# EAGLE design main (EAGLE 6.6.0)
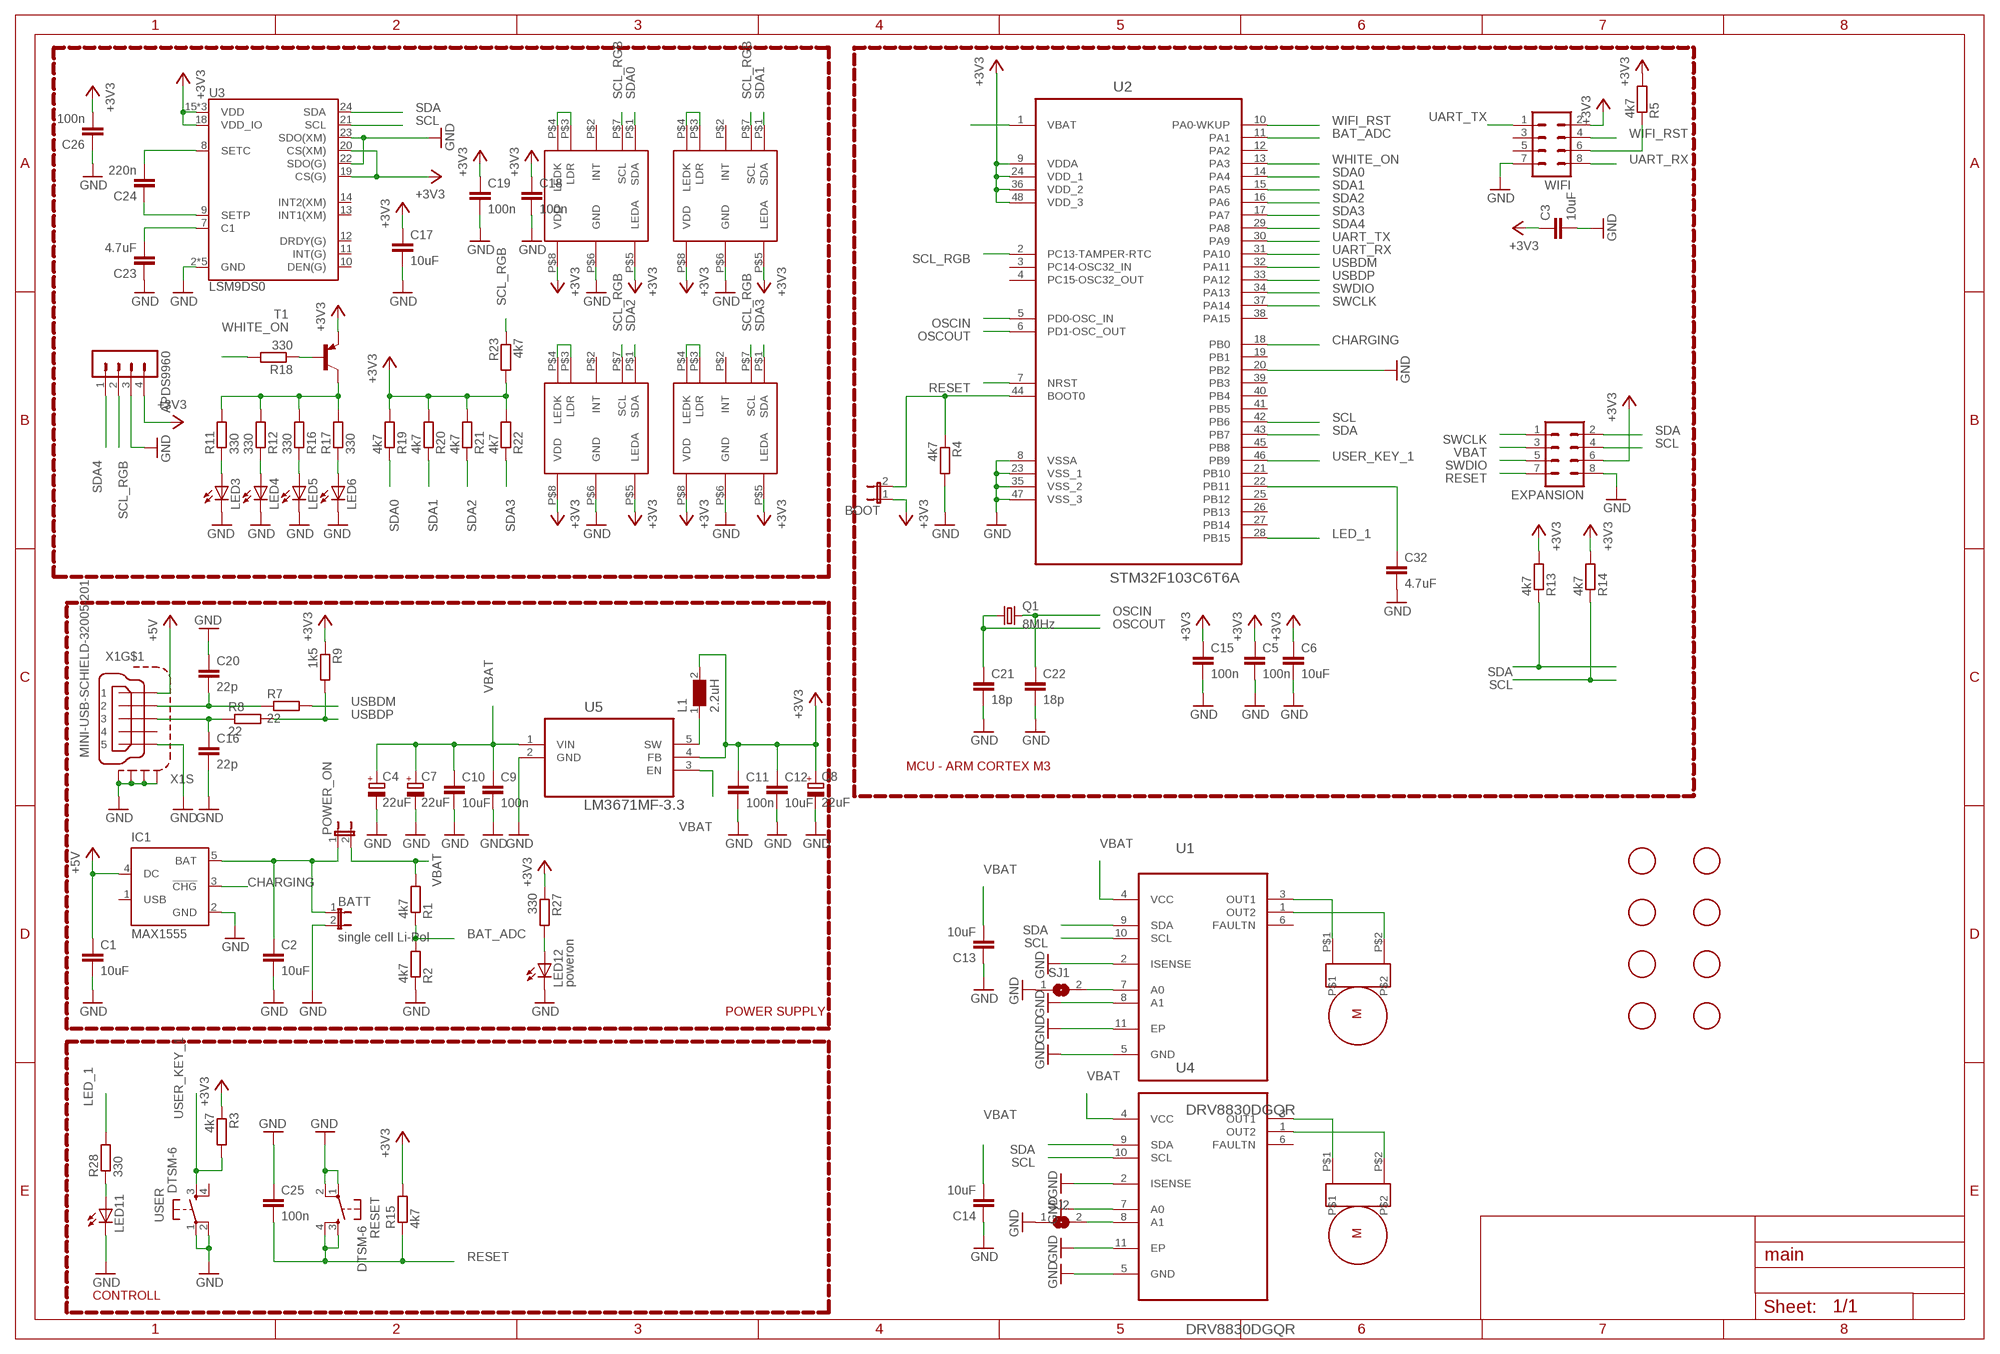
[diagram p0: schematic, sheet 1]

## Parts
APDS9960  MA04-1  [MA04-1]
BATT  single cell Li-Pol  JP1E  [JP1]
BOOT  JP1E  [JP1]
C1  10uF  C-EUC0805  [C0805]
C2  10uF  C-EUC0805  [C0805]
C3  10uF  C-EUC0805  [C0805]
C4  22uF  CPOL-EU153CLV-0505  [153CLV-0505]
C5  100n  C-EUC0805  [C0805]
C6  10uF  C-EUC0805  [C0805]
C7  22uF  CPOL-EU153CLV-0505  [153CLV-0505]
C8  22uF  CPOL-EU153CLV-0505  [153CLV-0505]
C9  100n  C-EUC0805  [C0805]
C10  10uF  C-EUC0805  [C0805]
C11  100n  C-EUC0805  [C0805]
C12  10uF  C-EUC0805  [C0805]
C13  10uF  C-EUC0805  [C0805]
C14  10uF  C-EUC0805  [C0805]
C15  100n  C-EUC0805  [C0805]
C16  22p  C-EUC0805  [C0805]
C17  10uF  C-EUC0805  [C0805]
C18  100n  C-EUC0805  [C0805]
C19  100n  C-EUC0805  [C0805]
C20  22p  C-EUC0805  [C0805]
C21  18p  C-EUC0805  [C0805]
C22  18p  C-EUC0805  [C0805]
C23  4.7uF  C-EUC0805  [C0805]
C24  220n  C-EUC0805  [C0805]
C25  100n  C-EUC0805  [C0805]
C26  100n  C-EUC0805  [C0805]
C32  4.7uF  C-EUC0805  [C0805]
EXPANSION  MA04-2  [MA04-2]
IC1  MAX1555  [SOT23-5L]
L1  2.2uH  WE-LQ-744032002_M  [WE-LQ_M]
LED3  LEDCHIPLED_1206  [CHIPLED_1206]
LED4  LEDCHIPLED_1206  [CHIPLED_1206]
LED5  LEDCHIPLED_1206  [CHIPLED_1206]
LED6  LEDCHIPLED_1206  [CHIPLED_1206]
LED11  LEDCHIPLED_1206  [CHIPLED_1206]
LED12  poweron  LEDCHIPLED_1206  [CHIPLED_1206]
POWER_ON  JP1E  [JP1]
Q1  8MHz  CRYSTALCTS406  [CTS406]
R1  4k7  R-EU_M0805  [M0805]
R2  4k7  R-EU_M0805  [M0805]
R3  4k7  R-EU_M1206  [M1206]
R4  4k7  R-EU_M0805  [M0805]
R5  4k7  R-EU_M0805  [M0805]
R7  22  R-EU_M0805  [M0805]
R8  22  R-EU_M0805  [M0805]
R9  1k5  R-EU_M0805  [M0805]
R11  330  R-EU_M0805  [M0805]
R12  330  R-EU_M0805  [M0805]
R13  4k7  R-EU_M0805  [M0805]
R14  4k7  R-EU_M0805  [M0805]
R15  4k7  R-EU_M0805  [M0805]
R16  330  R-EU_M0805  [M0805]
R17  330  R-EU_M0805  [M0805]
R18  330  R-EU_M0805  [M0805]
R19  4k7  R-EU_M0805  [M0805]
R20  4k7  R-EU_M0805  [M0805]
R21  4k7  R-EU_M0805  [M0805]
R22  4k7  R-EU_M0805  [M0805]
R23  4k7  R-EU_M0805  [M0805]
R27  330  R-EU_M0805  [M0805]
R28  330  R-EU_M0805  [M0805]
RESET  DTSM-6  [DTSM-6]
SJ1  SJ  [SJ]
SJ2  SJ  [SJ]
T1  BC857A-PNP-SOT23-BEC  [SOT23-BEC]
U1  DRV8830DGQR  [SOP65P640X110-15N]
U2  STM32F103C6T6A  [QFP50P900X900X160-48N]
U3  LSM9DS0  [LGA-24]
U4  DRV8830DGQR  [SOP65P640X110-15N]
U5  LM3671MF-3.3  [SOT95P284X122-5N]
U$1  APDS9950  [APDS9950]
U$2  APDS9950  [APDS9950]
U$3  APDS9950  [APDS9950]
U$4  APDS9950  [APDS9950]
U$5  MICRO_METAL_GEAR_MOTOR  [MICRO_METAL_GEAR_MOTOR]
U$6  MICRO_METAL_GEAR_MOTOR  [MICRO_METAL_GEAR_MOTOR]
U$9  FIDUCIAL  [FIDUCIAL_1MM]
U$10  FIDUCIAL  [FIDUCIAL_1MM]
U$11  FIDUCIAL  [FIDUCIAL_1MM]
U$12  FIDUCIAL  [FIDUCIAL_1MM]
U$13  FIDUCIAL  [FIDUCIAL_1MM]
U$14  FIDUCIAL  [FIDUCIAL_1MM]
U$15  FIDUCIAL  [FIDUCIAL_1MM]
U$16  FIDUCIAL  [FIDUCIAL_1MM]
USER  DTSM-6  [DTSM-6]
WIFI  MA04-2  [MA04-2]
X1  MINI-USB-SCHIELD-32005-201  [32005-201]

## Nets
+3V3: APDS9960.4 BOOT.1 C3.1 C5.1 C6.1 C8.+ C11.1 C12.1 C15.1 C17.1 C18.1 C19.1 C26.2 EXPANSION.6 L1.2 R3.1 R5.2 R9.1 R13.2 R14.2 R15.2 R19.2 R20.2 R21.2 R22.2 R23.2 R27.1 T1.E U2.9(VDDA) U2.24(VDD_1) U2.36(VDD_2) U2.48(VDD_3) U3.15(VDD) U3.16(VDD) U3.17(VDD) U3.18(VDD_IO) U3.19(CS(G)) U3.20(CS(XM)) U5.4(FB) U$1.P$5(LEDA) U$1.P$8(VDD) U$2.P$5(LEDA) U$2.P$8(VDD) U$3.P$5(LEDA) U$3.P$8(VDD) U$4.P$5(LEDA) U$4.P$8(VDD) WIFI.2
+5V: C1.1 IC1.4(DC) X1.1
BAT_ADC: R1.1 R2.2 U2.11(PA1)
CHARGING: IC1.3(!CHG) U2.18(PB0)
GND: APDS9960.3 BATT.2 C1.2 C2.2 C3.2 C4.- C5.2 C6.2 C7.- C8.- C9.2 C10.2 C11.2 C12.2 C13.1 C14.1 C15.2 C16.2 C17.2 C18.2 C19.2 C20.1 C21.2 C22.2 C23.1 C25.1 C26.1 C32.2 EXPANSION.8 IC1.2(GND) LED3.C LED4.C LED5.C LED6.C LED11.C LED12.C R2.1 R4.2 RESET.1 RESET.2 SJ1.1 SJ2.1 U1.2(ISENSE) U1.5(GND) U1.8(A1) U1.11(EP) U2.8(VSSA) U2.20(PB2) U2.23(VSS_1) U2.35(VSS_2) U2.47(VSS_3) U3.2(GND) U3.3(GND) U3.4(GND) U3.5(GND) U3.6(GND) U3.22(SDO(G)) U3.23(SDO(XM)) U4.2(ISENSE) U4.5(GND) U4.7(A0) U4.11(EP) U5.2(GND) U$1.P$6(GND) U$2.P$6(GND) U$3.P$6(GND) U$4.P$6(GND) USER.1 USER.2 WIFI.7 X1.5 X1.M1(S:S1) X1.M2(S:S2) X1.M3(S:S3) X1.M4(S:S4)
LED_1: R28.2 U2.28(PB15)
N$1: R5.1 WIFI.6
N$2: BATT.1 C2.1 IC1.5(BAT) POWER_ON.1
N$3: U1.1(OUT2) U$5.P$2
N$4: U1.3(OUT1) U$5.P$1
N$5: U4.1(OUT2) U$6.P$2
N$6: C23.2 U3.7(C1)
N$7: C24.2 U3.8(SETC)
N$8: U4.3(OUT1) U$6.P$1
N$9: L1.1 U5.5(SW)
N$13: C24.1 U3.9(SETP)
N$14: C32.1 U2.22(PB11)
N$15: LED3.A R11.1
N$16: BOOT.2 R4.1 U2.44(BOOT0)
N$17: U$1.P$3(LDR) U$1.P$4(LEDK)
N$18: U$2.P$3(LDR) U$2.P$4(LEDK)
N$19: U$3.P$3(LDR) U$3.P$4(LEDK)
N$20: U$4.P$3(LDR) U$4.P$4(LEDK)
N$21: SJ1.2 U1.7(A0)
N$22: LED4.A R12.1
N$23: LED12.A R27.2
N$24: LED5.A R16.1
N$25: LED6.A R17.1
N$26: R11.2 R12.2 R16.2 R17.2 T1.C
N$27: R18.1 T1.B
N$28: SJ2.2 U4.8(A1)
N$33: LED11.A R28.1
N$55: C20.2 R7.1 X1.2
N$56: C16.1 R8.1 X1.3
NC: U2.1(VBAT)
OSCIN: C22.1 Q1.3 U2.5(PD0-OSC_IN)
OSCOUT: C21.1 Q1.1 U2.6(PD1-OSC_OUT)
RESET: C25.2 EXPANSION.7 R15.1 RESET.3 RESET.4 U2.7(NRST)
SCL: EXPANSION.4 R14.1 U1.10(SCL) U2.42(PB6) U3.21(SCL) U4.10(SCL)
SCL_RGB: APDS9960.2 R23.1 U2.2(PC13-TAMPER-RTC) U$1.P$7(SCL) U$2.P$7(SCL) U$3.P$7(SCL) U$4.P$7(SCL)
SDA: EXPANSION.2 R13.1 U1.9(SDA) U2.43(PB7) U3.24(SDA) U4.9(SDA)
SDA0: R19.1 U2.14(PA4) U$1.P$1(SDA)
SDA1: R20.1 U2.15(PA5) U$2.P$1(SDA)
SDA2: R21.1 U2.16(PA6) U$3.P$1(SDA)
SDA3: R22.1 U2.17(PA7) U$4.P$1(SDA)
SDA4: APDS9960.1 U2.29(PA8)
SWCLK: EXPANSION.1 U2.37(PA14)
SWDIO: EXPANSION.5 U2.34(PA13)
UART_RX: U2.31(PA10) WIFI.8
UART_TX: U2.30(PA9) WIFI.1
USBDM: R7.2 U2.32(PA11)
USBDP: R8.2 R9.2 U2.33(PA12)
USER_KEY_1: R3.2 U2.46(PB9) USER.3
VBAT: C4.+ C7.+ C9.1 C10.1 C13.2 C14.2 EXPANSION.3 POWER_ON.2 R1.2 U1.4(VCC) U4.4(VCC) U5.1(VIN) U5.3(EN)
WHITE_ON: R18.2 U2.13(PA3)
WIFI_RST: U2.10(PA0-WKUP) WIFI.4
Unconnected: IC1.1(USB) U1.6(FAULTN) U2.3(PC14-OSC32_IN) U2.4(PC15-OSC32_OUT) U2.12(PA2) U2.19(PB1) U2.21(PB10) U2.25(PB12) U2.26(PB13) U2.27(PB14) U2.38(PA15) U2.39(PB3) U2.40(PB4) U2.41(PB5) U2.45(PB8) U3.10(DEN(G)) U3.11(INT(G)) U3.12(DRDY(G)) U3.13(INT1(XM)) U3.14(INT2(XM)) U4.6(FAULTN) U$1.P$2(INT) U$2.P$2(INT) U$3.P$2(INT) U$4.P$2(INT) USER.4 WIFI.3 WIFI.5 X1.4

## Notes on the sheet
- MCU - ARM CORTEX M3
- POWER SUPPLY
- CONTROLL

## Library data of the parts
APDS9960 = con-lstb:MA04-1: PIN HEADER; OC_FARNELL: unknown; OC_NEWARK: unknown
BATT BOOT POWER_ON = jumper:JP1E: JUMPER
C1-C3 C5 C6 C9-C26 C32 = resistor:C-EU: CAPACITOR, European symbol
C4 C7 C8 = resistor:CPOL-EU: POLARIZED CAPACITOR, European symbol
EXPANSION WIFI = con-lstb:MA04-2: PIN HEADER; OC_FARNELL: unknown; OC_NEWARK: unknown
IC1 = maxim:MAX1555: Dual-Input USB/AC Adapter 1-Cell Li+ Battery Chargers Source: http://www.maxim-ic.com .. MAX1551-MAX1555.pdf; MF: MAXIM; MPN: MAX1555EZK+T; OC_FARNELL: 1628222; OC_NEWARK: 59J2761
L1 = WE-LQ:WE-LQ: SMD RF Inductor WE-LQ; MPN: 744032002; OC_FARNELL: 1800378; OC_NEWARK: 78R5670; PACKAGE: 1210; SUPPLIER: WURTH ELEKTRONIK
LED3-LED6 LED11 LED12 = led:LED: LED
Q1 = crystal:CRYSTAL: CRYSTAL; OC_FARNELL: unknown; OC_NEWARK: unknown
R1-R5 R7-R9 R11-R23 R27 R28 = resistor:R-EU_: RESISTOR, European symbol
RESET USER = switch-tact:DTSM-6
SJ1 SJ2 = jumper:SJ: SMD solder JUMPER
T1 = my_parts:*-PNP-: PNP Transistror
U1 U4 = my_parts:DRV8830DGQR: LOW-VOLTAGE MOTOR DRIVER WITH SERIAL INTERFACE; MPN: DRV8830DGQR; OC_FARNELL: 1863106; OC_NEWARK: 58T1482; PACKAGE: MSOP-10; SUPPLIER: TEXAS INSTRUMENTS
U2 = stm32f103_lqfp48:STM32F103C6T6A: MCU, 32BIT, 32K FLASH, 48LQFP; MPN: STM32F103C6T6A; OC_FARNELL: 1972391; OC_NEWARK: 72T2643; PACKAGE: 48LQFP; SUPPLIER: STMicroelectronics
U3 = main:LSM9DS0: LSM9DS0 3D Accelerometer, 3D Gyroscope, 3D Magnetomter Features: 3 acceleration channels, 3 angular rate channels, 3 magnetic field channels ±2/±4/±6/±8/±16 g linear acceleration full scale ±2/±4/±8/±12 gauss magnetic full scale ±245/±500/±2000 dps angular rate full scale 16-bit data output SPI /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
U5 = my_parts:LM3671MF-3.3: IC BUCK SYNC 3.3V 0.6A; MPN: LM3671MF-3.3; OC_FARNELL: 1685767; OC_NEWARK: 79K7838; PACKAGE: 5-SOT-23; SUPPLIER: NationalSemiconductor
U$1-U$4 = my_parts:APDS9950
U$5 U$6 = pololu:MICRO_METAL_GEAR_MOTOR
U$9-U$16 = adafruit:FIDUCIAL: For use by pick and place machines to calibrate the vision/machine, 1mm
X1 = con-cypressindustries:MINI-USB-SCHIELD-: MINI USB-B Conector Source: www.cypressindustries.com; OC_FARNELL: unknown; OC_NEWARK: unknown

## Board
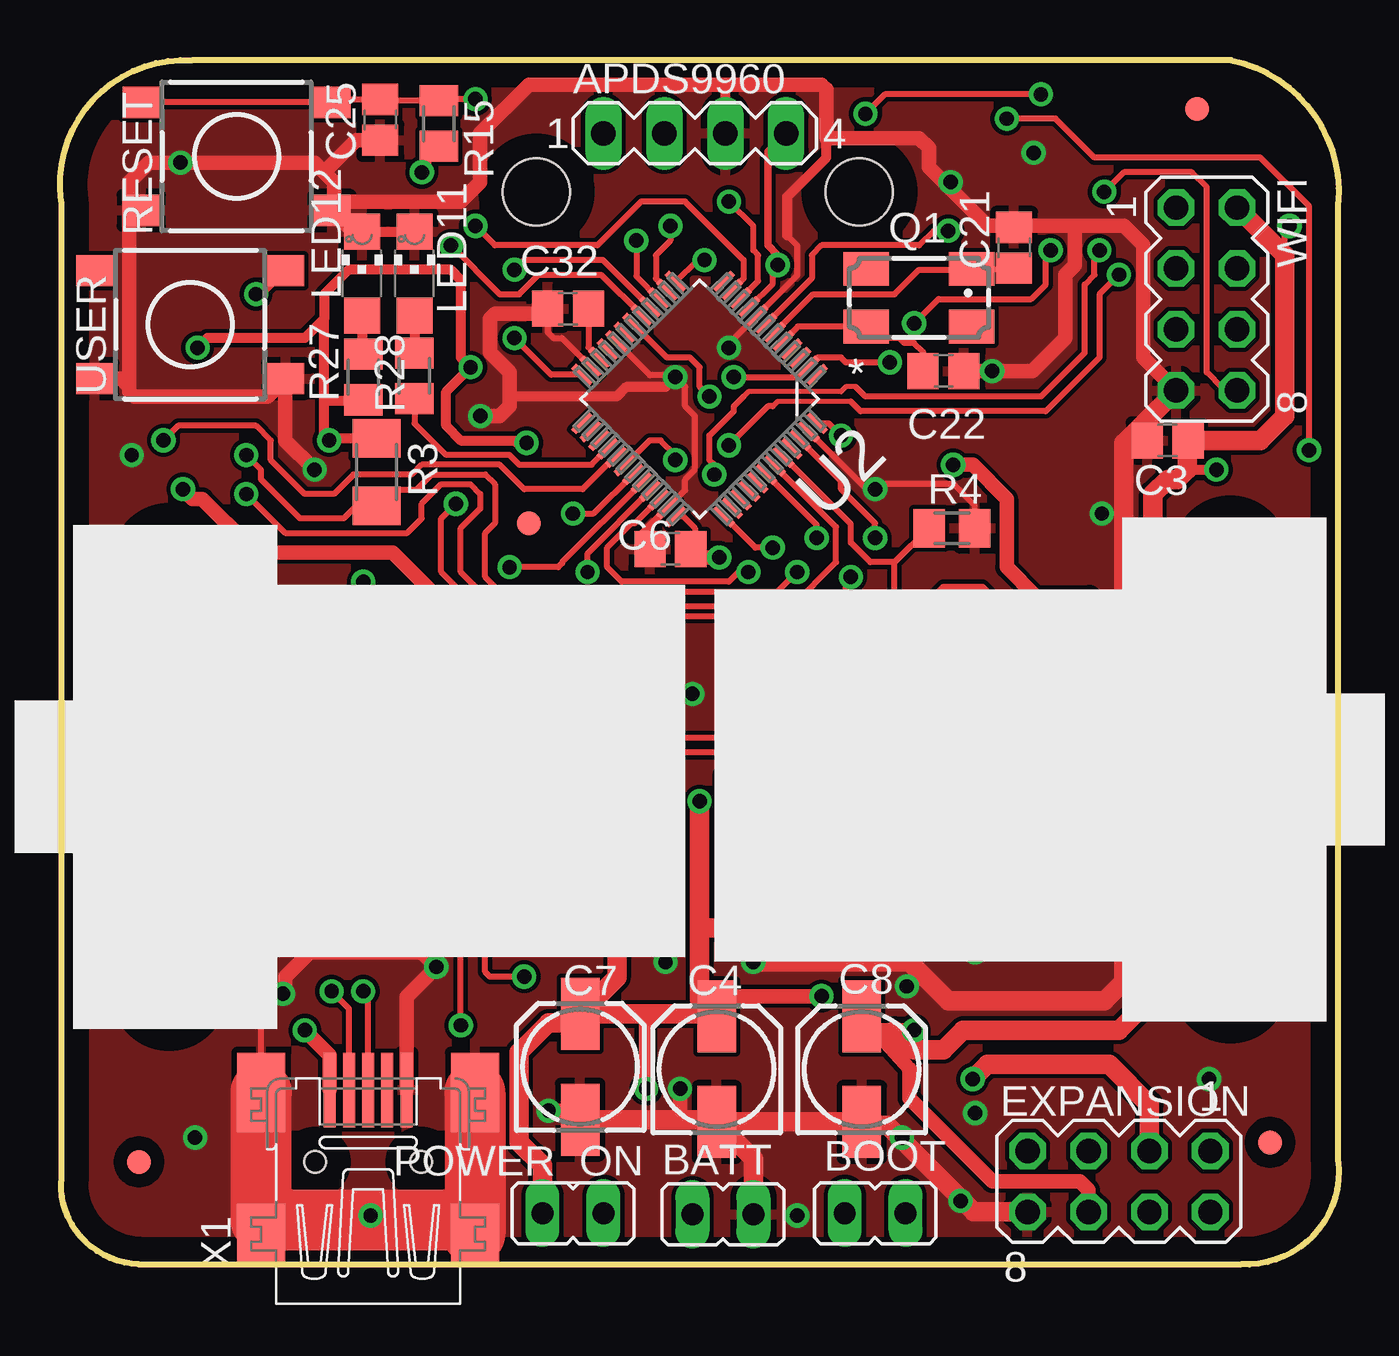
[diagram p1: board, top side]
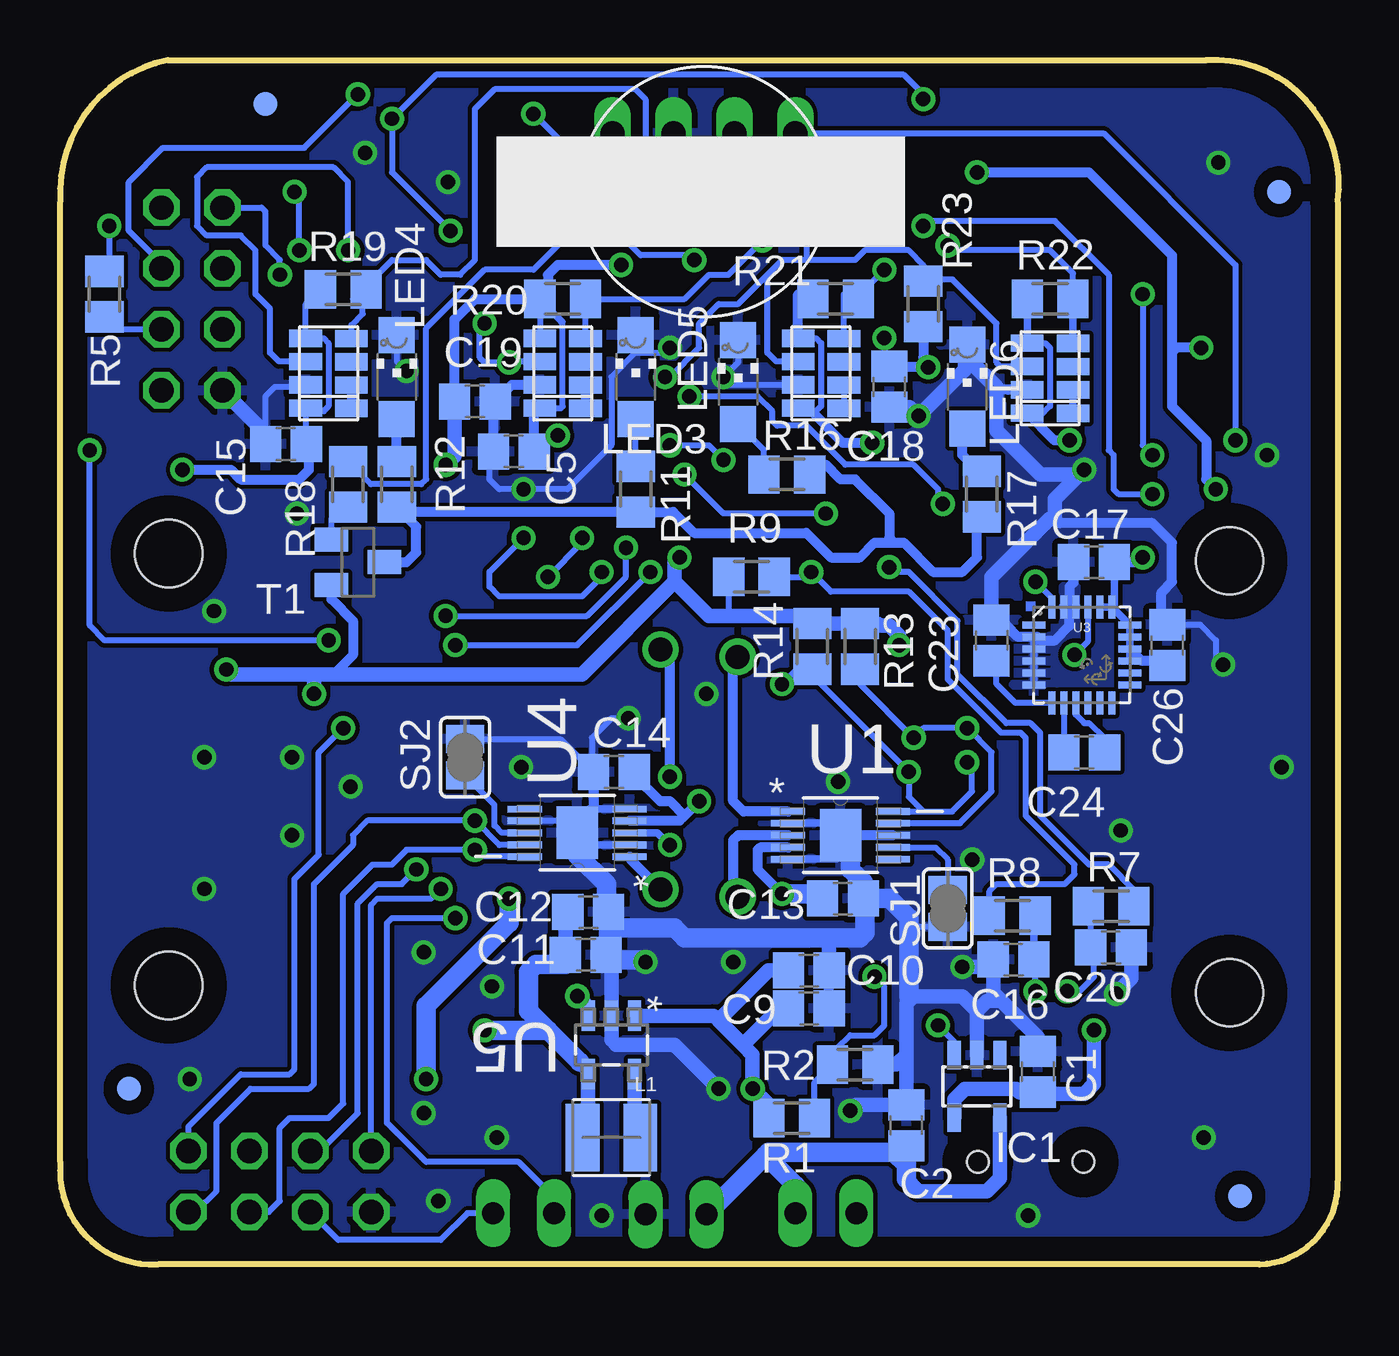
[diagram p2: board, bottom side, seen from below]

Size 53.3 x 50.2 mm. Coordinates in mm from the lower left corner, seen from the top.
Outline: 3.29,0 49.22,0 arc99 53.28,4.27 53.28,44.3 arc82 48.81,50.19 5.53,50.19 arc101 0.04,44.3 0.04,3.46 arc90 3.29,0
Copper layers (1*16): Top 0.035mm / dielectric 1.5mm / Bottom 0.035mm
Design rules "default *": minimum track width 7mil, minimum drill 24mil, track to track 7mil, track to pad 7mil, pad to pad 7mil, via to via 7mil, smd to smd 7mil, copper to edge 40mil, drill to drill 8mil, minimum pad ring 10mil, minimum via ring 8mil, stop-mask expansion 4mil, vias tented up to drill 0mil, thermal gap 10mil

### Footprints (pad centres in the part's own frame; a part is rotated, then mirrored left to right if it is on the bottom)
MA04-1 = drill 1.016 long: 1 -3.81,0; 2 -1.27,0; 3 1.27,0; 4 3.81,0
JP1 = drill 0.914 long: 1 0,-1.27; 2 0,1.27
C0805 = smd 1.3 x 1.5: 1 -0.85,0; 2 0.85,0
153CLV-0505 = smd 3 x 1.6: + 2.2,0; - -2.2,0
MA04-2 = drill 1.016 octagon: 1 -3.81,-1.27; 2 -3.81,1.27; 3 -1.27,-1.27; 4 -1.27,1.27; 5 1.27,-1.27; 6 1.27,1.27; 7 3.81,-1.27; 8 3.81,1.27
SOT23-5L = smd 0.55 x 1.2: 1 -0.95,-1.3; 2 0,-1.3; 3 0.95,-1.3; 4 0.95,1.3; 5 -0.95,1.3
WE-LQ_M = smd 1.4 x 2.8: 1 -1.2,0; 2 1.2,0
CHIPLED_1206 = smd 1.5 x 1.5: A 0,-1.75; C 0,1.75
CTS406 = smd 1.9 x 1.4: 1 -2.2,-1.2; 2 2.2,-1.2; 3 2.2,1.2; 4 -2.2,1.2
M0805 = smd 1.3 x 1.6: 1 -0.95,0; 2 0.95,0
M1206 = smd 1.6 x 2: 1 -1.4,0; 2 1.4,0
DTSM-6 = smd 1.55 x 1.3: 1 -3.975,2.25; 2 3.975,2.25; 3 -3.975,-2.25; 4 3.975,-2.25
SJ = smd 1.168 x 1.6: 1 -0.762,0; 2 0.762,0
SOT23-BEC = smd 1 x 1.4: B -0.95,-1.1; C 0,1.1; E 0.95,-1.1
SOP65P640X110-15N = smd 1.422 x 0.279: 1 -2.184,0.991; 2 -2.184,0.508; 3 -2.184,0; 4 -2.184,-0.508; 5 -2.184,-0.991; 6 2.184,-0.991; 7 2.184,-0.508; 8 2.184,0; 9 2.184,0.508; 10 2.184,0.991 | smd 1.727 x 2.184: 11 0,0
QFP50P900X900X160-48N = smd 1.041 x 0.279: 1 -4.166,2.743; 2 -4.166,2.261; 3 -4.166,1.753; 4 -4.166,1.245; 5 -4.166,0.762; 6 -4.166,0.254; 7 -4.166,-0.254; 8 -4.166,-0.762; 9 -4.166,-1.245; 10 -4.166,-1.753; 11 -4.166,-2.261; 12 -4.166,-2.743; 25 4.166,-2.743; 26 4.166,-2.261; 27 4.166,-1.753; 28 4.166,-1.245; 29 4.166,-0.762; 30 4.166,-0.254; 31 4.166,0.254; 32 4.166,0.762; 33 4.166,1.245; 34 4.166,1.753; 35 4.166,2.261; 36 4.166,2.743 | smd 0.279 x 1.041: 13 -2.743,-4.166; 14 -2.261,-4.166; 15 -1.753,-4.166; 16 -1.245,-4.166; 17 -0.762,-4.166; 18 -0.254,-4.166; 19 0.254,-4.166; 20 0.762,-4.166; 21 1.245,-4.166; 22 1.753,-4.166; 23 2.261,-4.166; 24 2.743,-4.166; 37 2.743,4.166; 38 2.261,4.166; 39 1.753,4.166; 40 1.245,4.166; 41 0.762,4.166; 42 0.254,4.166; 43 -0.254,4.166; 44 -0.762,4.166; 45 -1.245,4.166; 46 -1.753,4.166; 47 -2.261,4.166; 48 -2.743,4.166
LGA-24 = smd 0.954 x 0.29: 1 -2.002,1.25; 2 -2.002,0.75; 3 -2.002,0.25; 4 -2.002,-0.25; 5 -2.002,-0.75; 6 -2.002,-1.25; 13 2.002,-1.25; 14 2.002,-0.75; 15 2.002,-0.25; 16 2.002,0.25; 17 2.002,0.75; 18 2.002,1.25 | smd 0.29 x 0.954: 7 -1.25,-2.002; 8 -0.75,-2.002; 9 -0.25,-2.002; 10 0.25,-2.002; 11 0.75,-2.002; 12 1.25,-2.002; 19 1.25,2.002; 20 0.75,2.002; 21 0.25,2.002; 22 -0.25,2.002; 23 -0.75,2.002; 24 -1.25,2.002
SOT95P284X122-5N = smd 1.27 x 0.559: 1 -1.219,0.965; 2 -1.219,0; 3 -1.219,-0.965; 4 1.219,-0.965; 5 1.219,0.965
APDS9950 = smd 1.362 x 0.72: P$1 0.954,1.4; P$2 0.954,0.43; P$3 0.954,-0.54; P$4 0.954,-1.51; P$5 -0.954,-1.5; P$6 -0.954,-0.53; P$7 -0.954,0.44; P$8 -0.954,1.41
MICRO_METAL_GEAR_MOTOR = drill 1: P$1 -5,1; P$2 5,1 | hole 2.8: -9,21.5; 9,21.5
BALL_3/8 = hole 2.8: -6.35,0; 7.112,0
FIDUCIAL_1MM = smd 1 x 1: 1 0,0
32005-201 = smd 3.1 x 0.5: 1 3,1.6; 2 3,0.8; 3 3,0; 4 3,-0.8; 5 3,-1.6 | smd 2.5 x 2: M1 -3,-4.45; M2 -3,4.45 | smd 3.3 x 2: M3 2.9,4.45; M4 2.9,-4.45 | hole 0.9: 0,2.2; 0,-2.2

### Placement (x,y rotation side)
APDS9960  26.46,47.14 0 top
BATT  27.63,2.09 270 top
BOOT  33.98,2.14 90 top
C1  12.54,8.03 90 bottom
C2  18.03,5.79 90 bottom
C3  46.17,34.34 180 top
C4  27.37,8.13 90 top
C5  34.38,33.89 180 bottom
C6  25.44,29.82 180 top
C7  21.68,8.23 90 top
C8  33.42,8.13 90 top
C9  22.09,10.67 0 bottom
C10  22.09,12.25 0 bottom
C11  31.39,12.91 0 bottom
C12  31.29,14.68 0 bottom
C13  20.67,15.24 180 bottom
C14  30.22,20.53 0 bottom
C15  43.88,34.19 180 bottom
C16  13.56,12.7 180 bottom
C17  10.2,29.26 180 bottom
C18  18.74,36.58 270 bottom
C19  36.01,35.97 0 bottom
C20  9.49,13.21 180 bottom
C21  39.77,42.37 90 top
C22  36.82,37.24 0 top
C23  14.47,26.01 270 bottom
C24  10.61,21.34 180 bottom
C25  13.35,47.7 90 top
C26  7.16,25.81 270 bottom
C32  21.18,39.83 180 top
EXPANSION  44.14,3.46 180 top
IC1  15.08,7.42 180 bottom
L1  30.32,5.29 180 bottom
LED3  29.3,36.98 0 bottom
LED4  39.26,36.98 0 bottom
LED5  25.04,36.78 0 bottom
LED6  15.49,36.58 0 bottom
LED11  14.78,41.3 0 top
LED12  12.59,41.3 0 top
POWER_ON  21.38,2.14 90 top
Q1  35.81,40.29 180 top
R1  22.8,6.1 180 bottom
R2  20.16,8.33 180 bottom
R3  13.2,33.02 270 top
R4  37.18,30.69 0 top
R5  51.45,40.44 90 bottom
R7  9.49,14.94 0 bottom
R8  13.61,14.53 180 bottom
R9  24.48,28.65 0 bottom
R11  29.3,32.31 270 bottom
R12  39.26,32.51 270 bottom
R13  19.96,25.76 90 bottom
R14  21.94,25.76 90 bottom
R15  15.79,47.55 270 top
R16  23.01,32.92 0 bottom
R17  14.88,32.11 270 bottom
R18  41.29,32.51 90 bottom
R19  41.5,40.64 180 bottom
R20  32.35,40.24 180 bottom
R21  20.97,40.24 180 bottom
R22  12.03,40.24 180 bottom
R23  17.32,40.03 270 bottom
R27  12.64,36.98 90 top
R28  14.78,37.04 270 top
RESET  7.36,46.18 180 top
SJ1  16.3,14.84 90 bottom
SJ2  36.42,21.14 270 bottom
T1  40.89,29.26 270 bottom
U1  20.77,17.88 0 bottom
U2  26.66,36.07 225 top
U3  10.71,25.4 0 bottom
U4  31.74,17.99 180 bottom
U5  30.32,9.15 270 bottom
U$1  42.11,37.19 0 bottom
U$2  32.35,37.19 0 bottom
U$3  21.58,37.19 0 bottom
U$4  12.03,36.98 0 bottom
U$5  26.05,20.32 90 top
U$6  27.27,20.63 270 top
U$7  [BALL_3/8]  26.97,44.71 0 bottom
U$8  [LOGO_SMALL_BMP]  6.14,24.59 270 bottom
U$9  3.3,4.27 0 top
U$10  50.44,5.08 0 top
U$11  47.39,48.16 0 top
U$12  19.55,30.89 0 top
U$13  50.44,7.32 0 bottom
U$14  2.48,44.71 0 bottom
U$15  44.75,48.36 0 bottom
U$16  4.11,2.85 0 bottom
USER  5.43,39.17 180 top
WIFI  47.8,40.24 270 top
X1  12.85,4.27 90 top

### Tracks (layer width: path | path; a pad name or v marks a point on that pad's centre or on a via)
+3V3  (via drill 0.6)
  Top 0.254: 33.79,9.76 33.79,9.96 C8.+ | U2.36 25.96,31.19 26.46,30.69 26.46,29.99 C6.1 | U2.24 20.48,37.08 v18.94,38.61 | U2.48 32.04,35.06 v32.56,34.55 | U2.9 29.71,40.88 29.71,41.46 v29.91,41.66 | 51.05,42.06 51.05,43.08 v51.25,43.28 | R15.2 15.35,46.6 15.35,45.79 v15.08,45.52
  Top 0.305: v29.91,41.66 29.91,42.06 29.51,42.47 29.51,46.38 APDS9960.4
  Top 0.406: R27.1 12.59,35.98 11.03,35.98 11.02,35.97 | C6.1 26.71,29.62 | 11.39,34.18 v11.22,34.34 | 46.98,33.12 v48.2,33.12 | 19.04,34.24 v19.45,34.24 19.35,34.34 16.71,34.34 16.1,34.95 16.1,36.38 v17.11,37.39 16.71,37.8 16.71,41.05 16.3,41.46 12.03,41.46 11.02,40.44 11.02,39.42 | 8.48,29.97 8.58,29.87 | 11.02,39.42 10.2,38.61 6.14,38.61 v5.73,38.2 | 11.02,35.97 11.02,34.55 v11.22,34.34 | 11.02,35.97 11.02,39.42 | R3.1 11.3,34.42 v11.22,34.34
  Top 0.61: EXPANSION.6 42.87,3.1 42.51,3.46 38.85,3.46 35.4,6.91 35.4,8.15 C8.+ | v35.6,9.76 34.79,9.76 33.79,9.76 | v46.37,24.79 45.76,24.79 45.56,25 | v27.48,29.47 26.65,29.47 C6.1 | v37.23,33.33 38.04,33.33 39.46,31.9 39.46,29.06 40.68,27.84 42.92,27.84 43.33,27.43 43.33,24.39 v42.72,23.78 | 8.58,29.87 v8.17,29.47 7.97,29.47 | v18.33,25.81 18.13,26.01 17.52,26.01 13.86,29.67 8.78,29.67 8.48,29.97 7.87,29.97 5.94,31.9 5.53,31.9 v5.12,32.31
  Top 0.813: WIFI.2 51.05,42.06 51.05,35.36 50.03,34.34 C3.1 46.98,34.31 46.98,33.12 46.58,32.72 46.17,32.72 45.56,32.11 45.56,25 45.56,11.18 44.14,9.76 37.64,9.76 36.82,8.94 35.6,8.94 34.79,9.76
  Bottom 0.254: BOOT.1 36.31,2.14 37.43,1.02 41.7,1.02 EXPANSION.6 | U$4.P$8 12.22,38.39 12.03,38.2 12.03,35.77 12.44,35.36 12.86,35.36 U$4.P$5 | U$3.P$8 21.77,38.6 21.58,38.41 21.58,35.77 21.79,35.56 21.99,35.56 22.41,35.56 | 17.32,37.59 v17.11,37.39 | C26.2 6.95,25.15 | R9.1 25.43,27.22 25.24,27.03 | C15.1 43.06,34.22 U$1.P$5 42.93,35.56 42.31,35.56 42.11,35.77 42.11,38.41 42.3,38.6 U$1.P$8 43.06,40.03 R19.2 | U$2.P$8 R20.2 32.35,39.29 | U$2.P$5 32.43,35.69 32.35,35.77 32.35,39.29 | v18.94,38.61 18.94,37.63 | v32.56,34.55 32.87,34.55 C5.1 | 32.35,39.29 32.42,39.29 32.76,39.63 | v51.25,43.28 51.25,41.59 R5.2
  Bottom 0.305: C17.1 9.35,27.39 U3.19 | U3.15 U3.16 U3.17 U3.18 U3.19 | U3.20 U3.19 | U$4.P$8 R22.2
  Bottom 0.406: R13.2 19.23,26.71 | 22.26,27.03 R14.2 | 18.94,37.63 C18.1 | U$3.P$8 22.54,40.44 R21.2 | v11.22,34.34 11.84,34.34 U$4.P$5 | 6.74,25.15 6.95,25.15 8.21,25.15 U3.16 | v19.45,34.24 20.67,34.24 21.99,35.56 | U$3.P$5 22.41,35.56 | C5.1 33.53,35.46 U$2.P$5 | 18.57,37.59 C18.1 | R23.2 17.32,37.8 v17.11,37.39 18.7,37.39 C18.1 | C19.1 36.86,39.39 36.01,40.24 R20.2 32.96,40.58 32.96,41.25 32.56,41.66 v29.91,41.66 | T1.E 41.99,27.72 41.09,26.82 41.09,25.4 41.9,24.59 | v48.2,33.12 46.17,33.12 45.76,32.72 43.33,32.72 42.92,33.12 42.92,34.08 C15.1 | C17.1 8.37,29.26 v8.17,29.47 | v15.08,45.52 10.41,45.52 6.95,42.06 6.95,38 | v5.73,38.2 6.75,38.2 6.95,38 | 6.95,38 6.95,35.77 5.53,34.34 5.53,32.72 v5.12,32.31
  Bottom 0.61: L1.2 31.34,5.47 31.34,5.9 31.29,5.95 U5.4 31.29,8.08 31.64,8.44 32.35,9.15 | 32.24,12.51 C11.1 32.24,14.58 C12.1 | 27.68,28.45 31.54,24.59 41.9,24.59 42.51,24.59 | 42.51,24.59 46.17,24.59 v46.37,24.79 | v18.33,25.81 18.33,26.22 18.74,26.62 19.14,26.62 19.23,26.71 | R13.2 R14.2 | 22.26,27.03 25.24,27.03 26.26,27.03 27.68,28.45 | 27.68,28.45 27.68,29.26 v27.48,29.47 | C19.1 36.86,33.7 v37.23,33.33 | v42.72,23.78 42.72,24.39 42.51,24.59
  Bottom 0.813: 32.24,12.51 33.46,12.51 33.77,12.19 33.77,10.57 32.96,9.76 | 32.96,9.76 31.64,8.44 | v35.6,9.76 32.96,9.76
+5V  (via drill 0.6)
  Top 0.61: X1.1 11.25,8.71 v10.2,9.76
  Bottom 0.61: IC1.4 16.03,6.88 15.59,7.32 13.45,7.32 13.32,7.18 C1.1 12.48,7.11 10.61,7.11 10.2,7.52 v10.2,9.76
BAT_ADC  (via drill 0.6)
  Top 0.254: v19.35,11.99 17.93,11.99 17.72,12.19 17.72,13.21 16.91,14.02 16.91,23.78 17.32,24.18 19.14,24.18 20.16,25.2 20.16,27.23 19.96,27.43 18.13,27.43 16.71,28.86 16.71,30.69 17.52,31.5 17.52,32.11 17.11,32.51 15.89,32.51 15.08,31.7 15.08,31.09 14.47,30.48 9.39,30.48 v7.77,32.11 | v17.32,43.28 18.13,42.47 22.4,42.47 24.22,44.3 26.05,44.3 28.49,41.86 28.49,41.1 U2.11
  Bottom 0.254: R1.1 21.85,7.59 R2.2 21.11,9.01 20.91,9.01 20.36,9.55 19.35,9.55 18.94,9.96 18.94,11.58 v19.35,11.99 | v17.32,43.28 17.11,43.49 11.83,43.49 9.59,41.25 9.59,33.94 9.39,33.73 9.39,32.31 9.19,32.11 v7.77,32.11
CHARGING  (via drill 0.6)
  Top 0.254: 23.9,39.14 U2.18 25.29,37.8 26.26,37.8 26.66,37.39 26.66,36.58 v27.07,36.17 | v16.71,9.96 16.71,13.41 16.3,13.82 16.3,24.39 16.71,24.79 18.74,24.79 19.55,25.61 19.55,26.22 18.94,26.82 17.93,26.82 15.89,28.86 15.89,31.09 v16.5,31.7
  Bottom 0.254: v27.07,36.17 24.22,36.17 23.61,35.56 23.61,35.16 23.41,34.95 22.19,34.95 20.57,33.33 17.72,33.33 16.71,32.31 16.71,31.9 v16.5,31.7 | IC1.3 16.03,9.28 v16.71,9.96
GND  (via drill 0.6)
  Top 0.254: U2.23 20.93,38.61 20.57,38.61 20.33,38.85 C32.2 | 23.18,38.44 U2.20 24.59,37.06 25.57,37.06 v25.65,36.98 26.05,36.58 26.05,35.77 26.46,35.36 26.46,33.12 26.05,32.72 26.05,32.26 24.96,31.17 | U2.47 33.62,32.31 v33.98,32.31 34.18,32.51 37.23,32.51 38.13,31.62 R4.2 | v27.88,38.2 27.88,38.37 U2.8 30.73,41.21 30.73,42.47 30.32,42.88 | 17.25,1.22 X1.M1 | X1.M3 8.4,10.55 v9.29,11.28 | RESET.2 3.06,43.93 2.89,44.1
  Top 0.305: C6.2 24.19,30.4 24.96,31.17 U2.35
  Top 0.406: 12.56,43.08 LED12.C LED11.C | C3.2 44.75,34.34 44.34,33.94 | 18.74,36.38 18.94,36.17 23.21,36.17 23.61,36.58 25.24,36.58 v25.65,36.98 | APDS9960.3 27.73,48.92 27.48,49.18 | 30.32,42.88 30.32,44.5 31.95,46.13 31.95,46.94
  Top 0.61: v20.36,6.4 21.31,6.4 C7.- | v25.85,7.32 25.85,6.03 | v17.52,35.36 18.33,35.36 18.74,35.77 18.74,36.38 18.74,37.19 17.93,38 17.93,39.42 18.13,39.63 20.12,39.63 C32.2 | C22.2 v38.85,37.24 40.53,37.24 41.9,38.61 41.9,41.25 42.31,41.66 42.31,43.28 | 39.83,43.28 C21.2 | 39.83,43.28 38.65,43.28 36.21,45.72 36.21,46.54 35.81,46.94 31.95,46.94 31.95,48.97 31.74,49.18 27.48,49.18 19.55,49.18 17.52,47.14 17.52,45.11 16.71,44.3 11.7,44.3 RESET.1 | 39.83,43.28 42.31,43.28 | 42.31,43.28 44.34,43.28 45.15,42.47 45.15,37.8 WIFI.7 | X1.5 14.45,11.15 v15.69,12.4 15.08,13.01 10.41,13.01 9.39,11.99 9.39,11.38 v9.29,11.28 | 2.89,36.58 2.89,44.1 2.89,45.11 3.7,45.93 10.61,45.93 11.02,45.52 | USER.2 2.55,36.92 2.89,36.58 | 11.02,45.52 11.42,45.11 11.42,44.02 RESET.1 | 12.56,43.08 12.18,43.08 RESET.1 | C25.1 12.35,46.85 11.02,45.52 | 2.89,36.58 2.89,36.38 3.09,36.17 8.66,36.17 USER.1 9.39,36.91 9.39,34.34 v10.61,33.12
  Top 0.813: C7.- 25.85,6.03 27.27,6.03 C4.- | C4.- 32.66,5.93 | 32.66,5.93 C8.- | 27.68,5.63 C4.- | EXPANSION.8 38.09,2.19 34.49,5.79 32.79,5.79 32.66,5.93 | v28.9,12.6 35.4,12.6 37.03,10.98 43.53,10.98 44.34,11.79 44.34,33.94 44.34,34.24 WIFI.7 | BATT.2 28.9,4.41 C4.-
  Top 2.54: X1.M4 X1.M1 | 17.25,1.22 17.25,1.83 8.37,1.83 8.37,7.17 X1.M3
  Bottom 0.254: C15.2 44.73,36.19 44.34,36.58 43.14,36.58 U$1.P$6 | U$3.P$6 25.32,36.66 v25.65,36.98 25.04,37.59 LED5.C | LED3.C 29.3,38 | 29.3,38 30.32,36.98 30.32,34.14 32.15,32.31 v33.98,32.31 34.99,32.31 35.4,32.72 35.4,33.72 C5.2 | LED4.C 39.26,37.65 v38.85,37.24 | 29.3,38 28.09,38 v27.88,38.2 | v29.61,22.76 30.32,22.76 31.13,21.95 31.13,20.59 C14.1 32.44,21.9 SJ2.1 | v4.82,25 5.12,25.3 5.12,26.01 5.77,26.66 C26.1 7.23,26.66 7.4,26.82 | SJ1.1 17.77,14.07 17.93,14.23 | U4.7 32.25,18.49 U4.11
  Bottom 0.305: 20.26,17.38 20.36,17.48 | 20.36,17.48 U1.11 21.28,18.39 U1.2 | U1.5 20.95,16.89 20.47,17.38 20.36,17.48 | U4.2 31.23,17.48 U4.11 31.54,18.19 31.54,18.49 31.54,18.7 31.26,18.98 U4.5 | 11.22,29.43 C17.2 | 11.05,27.37 U3.22 | 11.42,27.24 U3.23 | U3.2 U3.3 U3.4 U3.5 U3.6
  Bottom 0.406: C14.1 31.07,18.96 31.54,18.49 | C23.1 14.23,26.62 13.86,26.62 13.39,26.15 U3.2 12.58,26.15 12.44,26.01 11.83,26.01 11.22,26.62 11.22,27.16 | 11.22,27.16 U3.23 11.22,27.65 11.22,28.25 11.05,28.41 C17.2 11.02,29.3 | 11.22,27.16 11.2,27.16 U3.22 | 13.78,36.45 U$4.P$6 14.35,36.45 15.59,37.7 15.49,37.8 LED6.C | 18.7,35.77 C18.2 | 7.4,26.66 7.4,26.82 7.4,28.01 6.95,28.45 6.95,30.08 7.77,30.89 11.63,30.89 11.83,31.09 | C9.2 C10.2 | U$2.P$6 34.47,36.66 C19.2 35.23,35.89 C5.2 | U1.8 U1.11
  Bottom 0.61: 20.12,6.44 v20.36,6.4 20.12,6.64 C2.2 18.03,8.74 | IC1.2 15.08,10.57 | 15.08,10.57 14.67,10.98 14.06,10.98 | 14.06,10.98 14.41,11.32 C16.2 14.71,12.4 v15.69,12.4 | v25.85,7.32 27.68,9.15 30.12,9.15 30.32,9.35 U5.2 30.32,12.69 C11.2 30.54,14.58 C12.2 | C23.1 14.47,28.65 12.03,31.09 11.83,31.09 11.83,31.9 v10.61,33.12 10.81,32.92 12.44,32.92 14.27,34.75 14.27,36.58 15.49,37.8 | 15.59,37.7 15.59,37.29 v17.52,35.36 17.89,35.73 C18.2 | C15.2 44.73,34.63 WIFI.7 | C10.2 21.24,13.55 21.18,13.62 | 15.08,10.57 15.69,11.18 17.72,11.18 | 17.72,11.18 17.93,11.18 | C1.2 12.54,9.45 14.06,10.98 | 18.03,8.74 18.03,10.87 17.72,11.18 | R2.1 18.43,8.33 18.03,8.74 | C20.1 8.64,11.93 v9.29,11.28
  Bottom 0.813: 20.47,17.38 20.36,17.27 20.36,16.46 19.82,15.92 C13.1 | C13.1 18.74,15.24 17.93,14.43 17.93,14.23 17.93,11.18 | C13.1 19.75,15.18 19.75,13.82 19.96,13.62 21.18,13.62 27.27,13.62 27.68,14.02 29.91,14.02 30.52,14.63 30.52,14.77 | U4.11 31.74,17.07 30.52,15.85 30.52,14.84 | 30.52,14.84 30.52,14.77 | 30.52,14.77 C12.2 | 30.32,12.69 28.99,12.69 v28.9,12.6 | 30.52,14.84 30.32,14.63 30.32,12.8
  other vias: 15.28,16.87 9.09,18.09 20.87,20.12 34.08,20.73 47.29,21.14 43.63,21.14 41.19,19.92 47.9,7.72 43.63,17.88 25.24,12.6 30.73,2.03 2.38,20.73 46.88,27.23 43.43,31.3 47.29,15.65 37.13,45.11 38.14,6.3 38.14,13.01 35.3,11.58 37.53,2.64 26.36,23.78 40.58,46.33 5.02,45.93 2.99,33.73 5.63,5.29 35.1,5.29 12.95,2.03
  pour Bottom: -6.46,55.48 58.97,55.48 58.97,-7.11 -6.46,-7.11
  pour Top: -2.6,52.43 62.63,52.43 62.63,-18.29 -2.6,-18.29
LED_1
  Top 0.254: R28.2 14.78,35.05 16.1,33.73 18.74,33.73 19.14,33.33 22.16,33.33 U2.28
N$1
  Bottom 0.254: WIFI.6 50.93,38.97 R5.1
N$2
  Bottom 0.61: IC1.5 14.13,3.59 14.67,3.05 17.52,3.05 18.03,3.56 C2.1
  Bottom 0.813: 23.89,4.55 23.77,4.68 18.53,4.68 18.03,4.17 18.03,3.56 | 23.89,4.55 BATT.1 | POWER_ON.1 22.65,3.3 23.89,4.55
N$3
  Bottom 0.406: U1.1 24.81,18.87 25.24,19.31 25.24,25.14 U$5.P$2
N$4
  Bottom 0.406: U1.3 25.04,17.88 25.24,17.68 25.24,15.51 U$5.P$1
N$5
  Bottom 0.406: U$6.P$2 29.49,16.85 29.49,16.93 U4.1
N$6
  Bottom 0.254: U3.7 13.48,23.4 14.27,24.18 14.27,24.96 C23.2
N$7
  Bottom 0.254: 11.46,21.75 C24.2 U3.8
N$8  (via drill 0.6)
  Top 0.406: v27.88,17.48 v27.88,20.32
  Bottom 0.305: U4.3 28.39,17.99 v27.88,17.48
  Bottom 0.406: v27.88,20.32 27.88,25.24 U$6.P$1
N$9
  Bottom 0.61: U5.5 29.36,5.52 L1.1
N$13
  Bottom 0.254: C24.1 9.76,21.91 10.41,22.56 10.61,22.56 10.96,22.91 U3.9
N$14
  Top 0.254: C32.1 22.03,38.23 U2.22
N$15
  Bottom 0.254: R11.1 LED3.A
N$16  (via drill 0.6)
  Top 0.254: v36.82,14.43 36.82,14.84 36.42,15.24 36.42,16.46 36.82,16.87 36.82,21.34 34.79,23.37 34.79,29.25 R4.1 34.79,29.26 33.77,29.26 32.96,30.08 32.96,30.85 U2.44
  Bottom 0.254: BOOT.2 32.71,2.8 34.18,4.27 38.04,4.27 39.67,5.9 39.67,14.23 39.46,14.43 v36.82,14.43
N$17
  Bottom 0.406: U$1.P$3 U$1.P$4
N$18
  Bottom 0.406: U$2.P$3 U$2.P$4
N$19
  Bottom 0.254: U$3.P$3 U$3.P$4
N$20
  Bottom 0.305: U$4.P$3 U$4.P$4
N$21
  Bottom 0.254: U1.7 16.81,17.38 16.3,16.87 SJ1.2
N$22
  Bottom 0.406: R12.1 LED4.A
N$23
  Top 0.406: LED12.A 12.59,37.99 R27.2
N$24
  Bottom 0.254: R16.1 23.96,33.95 LED5.A
N$25
  Bottom 0.254: 14.88,34.22 LED6.A
  Bottom 0.406: R17.1 15.01,33.06 15.69,33.73 15.69,34.63 LED6.A
N$26
  Bottom 0.406: T1.C 38.85,29.26 38.45,29.67 38.45,30.75 R12.2 39.06,31.36 R11.2 27.74,31.36 26.87,30.48 22.19,30.48 21.18,29.47 19.96,29.47 19.35,30.08 18.53,30.08 | 15.01,31.3 R17.2 15.08,30.95 15.08,29.47 15.69,28.86 16.91,28.86 18.13,30.08 18.53,30.08 | R16.2 21.38,33.33 20.77,32.72 20.16,32.72 18.74,31.3 18.74,30.28 18.53,30.08
N$27
  Bottom 0.254: T1.B 41.99,31.07 R18.1
N$28
  Bottom 0.254: U4.8 34.89,17.99 35.2,18.29 35.2,19.15 SJ2.2
N$33
  Top 0.406: LED11.A R28.1
N$55  (via drill 0.6)
  Top 0.254: X1.2 12.05,10.66 v11.32,11.38
  Bottom 0.254: R7.1 10.34,14.84 C20.2 10.2,13.07 10.2,11.99 10.81,11.38 v11.32,11.38
N$56  (via drill 0.6)
  Top 0.254: X1.3 12.85,11.18 v12.64,11.38
  Bottom 0.254: v12.64,11.38 12.64,12.64 C16.1
  Bottom 0.305: C16.1 12.71,14.48 R8.1
OSCIN
  Top 0.254: Q1.3 30.76,39.09 U2.5 | 33.68,39.02 Q1.3 | C22.1 35.97,38.04 35.6,38.41 35.2,38.41 34.99,38.61 34.08,38.61 Q1.3
OSCOUT
  Top 0.254: Q1.1 37.67,41.49 | U2.6 31.39,40.44 34.79,40.44 35.81,41.46 37.98,41.46 Q1.1 | Q1.1 39.74,41.49 C21.1
RESET  (via drill 0.6)
  Top 0.254: v37.43,15.65 37.43,22.35 35.81,23.98 35.81,27.23 36.82,28.25 38.45,28.25 40.89,25.81 41.9,25.81 v42.11,26.01 | v52.06,33.94 52.06,44.1 50.03,46.13 43.12,46.13 41.5,47.75 v39.46,47.75 | v37.03,43.08 36.42,43.08 35.81,42.47 31.74,42.47 31.34,42.06 31.34,41.1 U2.7 | RESET.4 RESET.3 11.46,48.55 C25.2 13.41,48.5 R15.1 15.86,48.57 v17.32,48.57
  Bottom 0.254: EXPANSION.7 40.33,14.99 40.07,15.24 37.84,15.24 v37.43,15.65 | v42.11,26.01 51.45,26.01 52.06,26.62 v52.06,33.94 | v37.03,43.08 39.46,45.52 v39.46,47.75 37.64,49.58 18.13,49.58 17.32,48.77 v17.32,48.57
SCL  (via drill 0.6)
  Top 0.254: v36.01,17.27 30.52,17.27 29.1,18.7 29.1,20.32 28.09,21.34 18.74,21.34 v17.93,20.53 | v11.02,25.4 v15.49,20.93 | v23.21,24.18 23.21,26.01 24.22,27.03 32.56,27.03 32.76,27.23 32.76,28.45 v32.96,28.65 | v31.54,30.28 31.54,30.83 U2.42
  Bottom 0.254: EXPANSION.4 44.6,2.19 44.14,2.64 44.14,5.69 43.73,6.1 42.11,6.1 41.5,6.71 41.5,15.45 40.28,16.66 39.46,16.66 38.85,17.27 v36.01,17.27 35.73,17 U4.10 | U3.21 10.46,25.96 v11.02,25.4 | U1.10 17.32,18.87 | 17.32,18.87 16.12,18.87 15.28,19.71 15.28,20.73 v15.49,20.93 | 17.32,18.87 17.93,19.48 v17.93,20.53 21.94,24.54 R14.1 22.58,24.81 v23.21,24.18 | v31.54,30.28 31.54,30.08 v32.96,28.65
SCL_RGB  (via drill 0.6)
  Top 0.254: v34.59,37.59 32.76,37.59 32.56,37.8 31.59,37.8 U2.2 30.77,36.98 v28.09,36.98 | v35.6,39.22 36.62,40.24 40.48,40.24 41.09,40.85 41.09,42.06 v41.29,42.27
  Bottom 0.254: U$4.P$7 14.1,37.42 14.27,37.59 14.27,39.22 16.1,41.05 17.25,41.05 R23.1 | U$3.P$7 23.45,37.63 23.82,38 23.82,41.25 | 17.79,41.46 R23.1 | R23.1 17.32,41.66 17.93,42.27 19.75,42.27 20.16,41.86 22.19,41.86 | 22.19,41.86 23.21,41.86 23.82,41.25 | U$2.P$7 34.55,37.63 v34.59,37.59 35.6,37.59 35.81,37.8 35.81,39.02 v35.6,39.22 | v28.09,36.98 27.88,36.98 26.66,38.2 26.66,39.22 25.85,40.03 25.04,40.03 23.82,41.25 | U$1.P$7 44.17,37.63 44.54,38 44.54,39.83 45.15,40.44 45.15,42.27 45.76,42.88 47.19,42.88 47.59,43.28 47.59,45.32 47.19,45.72 41.9,45.72 41.29,45.11 v41.29,42.27 | APDS9960.2 25.19,46.89 22.19,43.89 22.19,41.86
SDA  (via drill 0.6)
  Top 0.254: v36.01,18.49 35.4,18.49 34.79,17.88 30.73,17.88 29.71,18.9 29.71,20.53 28.29,21.95 v17.72,21.95 19.55,23.78 19.96,23.78 22.6,26.42 22.8,26.42 23.82,27.43 30.52,27.43 32.35,29.26 32.35,30.74 U2.43 | v12.64,28.45 12.64,25.2 v15.49,22.35
  Bottom 0.254: EXPANSION.2 47.64,2.19 46.78,3.05 46.78,5.9 45.36,7.32 42.92,7.32 42.72,7.52 42.72,15.85 41.09,17.48 41.09,17.88 40.48,18.49 v36.01,18.49 34.99,17.48 U4.9 | U3.24 11.96,27.77 v12.64,28.45 | v15.49,22.35 17.32,22.35 v17.72,21.95 19.96,24.18 R13.1 | U1.9 15.79,18.39 14.47,19.71 14.47,21.34 v15.49,22.35 | 15.28,22.15 v15.49,22.35
SDA0  (via drill 0.6)
  Top 0.254: v25.44,43.28 25.44,42.67 24.83,42.06 24.83,41.1 U2.14
  Bottom 0.254: U$1.P$1 41.16,39.15 40.68,39.63 40.68,40.51 R19.1 40.95,40.24 41.09,40.24 39.46,41.86 38.04,41.86 37.43,41.25 36.62,41.25 36.01,41.86 36.01,48.16 35.2,48.97 29.3,48.97 28.9,48.57 28.9,45.52 28.49,45.11 26.46,45.11 25.44,44.1 v25.44,43.28 25.44,43.08
SDA1  (via drill 0.6)
  Top 0.254: v24.02,42.67 24.02,41.19 U2.15
  Bottom 0.254: U$2.P$1 R20.1 | R20.1 | R20.1 27.28,40.23 26.26,41.25 25.44,41.25 24.63,42.06 v24.02,42.67
SDA2  (via drill 0.6)
  Top 0.254: U2.16 22.63,41.86 19.35,41.86 v18.94,41.46
  Bottom 0.254: U$3.P$1 20.63,40.44 R21.1 20.02,40.37 v18.94,41.46
SDA3  (via drill 0.6)
  Top 0.254: U2.17 22.56,41.25 19.96,41.25 19.14,40.44 18.33,40.44 v16.3,42.47
  Bottom 0.254: R22.1 11.08,41.31 12.03,42.27 16.1,42.27 v16.3,42.47
  Bottom 0.305: U$4.P$1 R22.1
SDA4  (via drill 0.6)
  Top 0.254: U2.29 23.14,33.66 21.79,32.31 19.35,32.31 18.33,33.33 15.08,33.33 14.67,32.92 12.24,32.92 11.42,32.11 10.2,32.11 8.78,33.53 8.78,34.34 8.17,34.95 4.92,34.95 v4.31,34.34
  Bottom 0.254: APDS9960.1 9.8,47.14 4.31,41.66 v4.31,34.34
SWCLK  (via drill 0.6)
  Top 0.254: v41.5,22.35 41.5,24.18 38.45,27.23 38.25,27.23 38.04,27.43 37.64,27.43 v37.23,27.03 | v29.71,29.87 28.98,29.87 U2.37
  Bottom 0.254: EXPANSION.1 47.95,5.74 45.76,7.93 43.73,7.93 43.53,8.13 43.53,16.06 42.51,17.07 42.51,21.34 v41.5,22.35 | v37.23,27.03 31.34,27.03 29.71,28.65 v29.71,29.87
SWDIO  (via drill 0.6)
  Top 0.254: v28.69,28.86 28.29,28.86 27.88,28.45 23.41,28.45 22.8,29.06 22.8,29.87 23.82,30.89 23.96,30.89 U2.34 | v38.45,16.46 38.45,22.56 36.62,24.39 36.62,25.61 v36.82,25.81
  Bottom 0.254: EXPANSION.5 42.46,4.73 40.89,6.3 40.89,15.04 40.07,15.85 39.06,15.85 v38.45,16.46 | v28.69,28.86 31.74,25.81 v36.82,25.81
UART_RX  (via drill 0.6)
  Top 0.203: 33.17,36.58 32.76,36.58 32.56,36.38 28.69,36.38 28.49,36.17
  Top 0.254: WIFI.8 49.07,36.53 48.46,36.53 47.8,37.19 47.8,44.91 47.19,45.52 44.34,45.52 v43.53,44.71 | U2.31 22.25,31.3 v21.38,31.3 | 33.17,36.58 33.57,36.17 40.89,36.17 42.72,38 42.72,40.85 43.12,41.25 43.12,42.06 v43.33,42.27 | v27.27,32.92 27.27,33.33 27.07,33.53 27.07,34.55 28.09,35.56 28.09,35.77 28.49,36.17
  Bottom 0.254: v21.38,31.3 25.65,31.3 v27.27,32.92 | v43.33,42.27 43.33,44.5 v43.53,44.71
UART_TX  (via drill 0.6)
  Top 0.203: 32.96,35.97 29.91,35.97 29.71,35.77
  Top 0.254: 32.96,35.97 33.37,35.56 41.09,35.56 43.33,37.8 43.33,40.44 v44.14,41.25 | v25.65,33.53 25.65,33.73 25.04,34.34 24.58,34.34 U2.30 | 29.71,35.77 29.51,35.77 v27.88,34.14
  Bottom 0.254: WIFI.1 44.9,44.05 44.75,43.89 44.75,42.47 44.14,41.86 v44.14,41.25 | v27.88,34.14 26.26,34.14 v25.65,33.53
USBDM  (via drill 0.6)
  Top 0.254: U2.32 20.93,29.26 20.93,29.22 20.77,29.06 v18.74,29.06
  Bottom 0.254: R7.2 8.54,15.61 9.59,16.66 10.41,16.66 12.44,18.7 12.44,22.15 12.85,22.56 13.86,22.56 15.89,24.59 15.89,26.82 17.93,28.86 18.53,28.86 v18.74,29.06
USBDP  (via drill 0.6)
  Top 0.254: v21.99,28.86 21.99,29.64 U2.33
  Bottom 0.254: R8.2 14.56,15.56 14.27,15.85 11.42,15.85 11.02,16.26 11.02,16.66 13.05,18.7 13.05,21.95 13.25,22.15 14.06,22.15 16.3,24.39 16.3,26.42 17.93,28.04 21.18,28.04 v21.99,28.86 22.19,28.65 R9.2
USER_KEY_1  (via drill 0.6)
  Top 0.254: v30.73,28.86 29.91,28.04 18.33,28.04 17.72,28.65 17.72,30.48 18.13,30.89 18.13,32.51 17.72,32.92 15.49,32.92 14.84,32.28 13.85,32.28 R3.2 13.12,31.7 12.44,31.7 11.83,31.09 10,31.09 8.37,32.72 8.37,33.12 v7.77,33.73 | v33.98,30.28 33.98,30.89 32.56,32.31 32.56,32.66 U2.46 | v8.17,40.44 8.42,40.44 USER.3
  Bottom 0.254: v30.73,28.86 30.73,28.65 31.54,27.84 34.99,27.84 35.4,28.25 35.4,28.86 v33.98,30.28 | v8.17,40.44 8.17,34.14 v7.77,33.73
VBAT  (via drill 0.6)
  Top 0.61: v24.43,7.32 24.43,10.23 24.63,10.43 | v31.74,11.18 28.22,11.18 C4.+
  Top 0.813: C7.+ 21.31,10.06 20.36,10.06 19.14,8.84 19.14,5.08 20.11,4.12 POWER_ON.2 | C7.+ 24.63,10.43 27.27,10.43 C4.+ 26.66,11.04 26.66,13.82 | v26.66,19.31 26.66,13.82 | v23.21,15.45 23.21,11.96 C7.+ | EXPANSION.3 45.41,6.66 43.73,8.33 38.65,8.33 v38.04,7.72 | v34.59,15.24 34.38,15.24 33.17,14.02 26.87,14.02 26.66,13.82
  Bottom 0.406: U1.4 24.12,17.38 24.22,17.27 24.22,16.46 v23.21,15.45 | U4.4 27.48,18.49 27.27,18.7 | 27.27,18.7 v26.66,19.31 | C14.2 29.37,20.39 28.29,19.31 27.88,19.31 27.27,18.7
  Bottom 0.61: R1.2 23.75,6.64 v24.43,7.32 24.43,8.74 24.83,9.15 | U5.1 26.05,10.37 25.85,10.16 | 25.85,10.16 24.83,9.15 | U5.3 31.29,10.72 v31.74,11.18 | C9.1 23.31,10.67 24.83,9.15 | C10.1 23.77,12.25 25.85,10.16
  Bottom 0.813: v23.21,15.45 21.72,15.45 C13.2 | v38.04,7.72 38.04,10.77 34.59,14.23 v34.59,15.24
WHITE_ON  (via drill 0.6)
  Top 0.254: v26.87,41.86 26.56,41.86 U2.13
  Bottom 0.254: v26.87,41.86 27.07,42.06 29.1,42.06 29.71,42.67 32.35,42.67 33.57,41.46 35.6,41.46 38.04,39.02 38.04,32.72 38.25,32.51 40.34,32.51 R18.2
WIFI_RST  (via drill 0.6)
  Top 0.254: v40.89,48.77 34.38,48.77 v33.57,47.96 | U2.10 29.1,40.99 29.1,42.06 28.9,42.27 28.9,43.28 v27.88,44.3
  Bottom 0.254: v40.89,48.77 43.12,46.54 49.01,46.54 50.44,45.11 50.44,43.08 49.07,41.71 WIFI.4 | v27.88,44.3 29.91,44.3 v33.57,47.96
(copper drawn outside any net)
  shapes: Bottom area x1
